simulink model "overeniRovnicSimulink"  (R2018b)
settings: Solver=ode4  StartTime=0.0  StopTime=5  FixedStep=1e-3  RelTol=1e-3
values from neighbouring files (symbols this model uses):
  b_0 = 0    [mainSkript_overeniRovnic.m]    (also in mainSkript_rovniceSystemu.m = (params.bp_0 + params.bn_0) / 2; mainSkript_simulaceLQG.m = (bn_0 + bp_0) / 2; mainSkript_LQGexperiment.m = (bn_0 + bp_0) / 2; mainSkript_LQGexperiment_integral.m = (bn_0 + bp_0) / 2)
  b_1 = params.b_1    [mainSkript_overeniRovnic.m]    (also in mainSkript_rovniceSystemu.m; mainSkript_kyvadlaNajednouOdhad.m; mainSkript_simulaceLQG.m; mainSkript_LQGexperiment.m)
  b_2 = params.b_2    [mainSkript_overeniRovnic.m]    (also in mainSkript_rovniceSystemu.m; mainSkript_kyvadlaNajednouOdhad.m; mainSkript_simulaceLQG.m; mainSkript_LQGexperiment.m)
  dtheta0_0 = 0    [mainSkript_overeniRovnic.m]
  dtheta0_1 = 0    [mainSkript_overeniRovnic.m]    (also in mainSkript_kyvadlaNajednouOdhad.m = filt * dth1(n_start-gl : n_start+gl))
  dtheta0_2 = 0    [mainSkript_overeniRovnic.m]    (also in mainSkript_kyvadlaNajednouOdhad.m = filt * dth2(n_start-gl : n_start+gl))
  g = 9.81    [mainSkript_overeniRovnic.m]    (also in mainSkript_rovniceSystemu.m; mainSkript_estimaceVozik.m; mainSkript_odhadKyvadlaZvlast.m; mainSkript_kyvadlaNajednouOdhad.m)
  I_1 = params.I_1    [mainSkript_overeniRovnic.m]    (also in mainSkript_rovniceSystemu.m; mainSkript_kyvadlaNajednouOdhad.m; mainSkript_simulaceLQG.m; mainSkript_LQGexperiment.m)
  I_2 = params.I_2    [mainSkript_overeniRovnic.m]    (also in mainSkript_rovniceSystemu.m; mainSkript_kyvadlaNajednouOdhad.m; mainSkript_simulaceLQG.m; mainSkript_LQGexperiment.m)
  L_1 = params.L_1    [mainSkript_overeniRovnic.m]    (also in mainSkript_rovniceSystemu.m; odhadovane_parametry.m = 0.228; mainSkript_kyvadlaNajednouOdhad.m; mainSkript_simulaceLQG.m)
  l_1 = params.l_1    [mainSkript_overeniRovnic.m]    (also in mainSkript_rovniceSystemu.m; odhadovane_parametry.m = 0.134; mainSkript_kyvadlaNajednouOdhad.m; mainSkript_simulaceLQG.m)
  l_2 = params.l_2    [mainSkript_overeniRovnic.m]    (also in mainSkript_rovniceSystemu.m; odhadovane_parametry.m = 0.112; mainSkript_kyvadlaNajednouOdhad.m; mainSkript_simulaceLQG.m)
  m = params.m_0    [mainSkript_estimaceVozik.m]    (also in mainSkript_odhadKyvadlaZvlast.m = params.m_2; mainSkript_modifikaceVozik.m = 1.437)
  m_0 = params.m_0    [mainSkript_overeniRovnic.m]    (also in mainSkript_rovniceSystemu.m; mainSkript_simulaceLQG.m; mainSkript_LQGexperiment.m; mainSkript_LQGexperiment_integral.m)
  m_1 = params.m_1    [mainSkript_overeniRovnic.m]    (also in mainSkript_rovniceSystemu.m; mainSkript_kyvadlaNajednouOdhad.m; mainSkript_simulaceLQG.m; mainSkript_LQGexperiment.m)
  m_2 = params.m_2    [mainSkript_overeniRovnic.m]    (also in mainSkript_rovniceSystemu.m; mainSkript_kyvadlaNajednouOdhad.m; mainSkript_simulaceLQG.m; mainSkript_LQGexperiment.m)
  N = N * Cref'    [mainSkript_simulaceLQG.m]    (also in mainSkript_tvorbaTrajektorii.m = 100; mainSkript_pocitaniTVLQR_simplified.m = floor( length(time) / krok ))
  theta0_0 = 0    [mainSkript_overeniRovnic.m]
  theta0_1 = 0.1    [mainSkript_overeniRovnic.m]
  theta0_2 = -0.6    [mainSkript_overeniRovnic.m]
undefined symbols (not defined in the file or in its folder): deg, DiscIntNeverNeededParam, kg, rad, s
libraries: mblibv1 x33, simulink x2
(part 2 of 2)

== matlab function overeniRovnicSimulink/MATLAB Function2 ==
function dx = PohybovaRceDIP_basic(y, u, g, m_0, m_1, m_2, I_1, I_2, l_1, l_2, L_1, b_0, b_1, b_2)
%PohybovaRceDIP_basic: Pohybova rovnice dvojiteho kyvadla

dx = zeros(6, 1); % definovani sloupcoveho vektoru derivaci stavu 

dx(1) = conj(y(4)); 
dx(2) = conj(y(5)); 
dx(3) = conj(y(6)); 
dx(4) = conj(y(6))*((b_2*(L_1^2*l_2*m_2^2*cos(y(3)) + I_1*l_2*m_2*cos(y(3)) - L_1^2*l_2*m_2^2*cos(y(2) - y(3))*cos(y(2)) + l_1^2*l_2*m_1*m_2*cos(y(3)) - L_1*l_1*l_2*m_1*m_2*cos(y(2) - y(3))*cos(y(2))))/(I_2*L_1^2*m_2^2 + I_2*l_1^2*m_1^2 + I_1*l_2^2*m_2^2 + I_1*I_2*m_0 + I_1*I_2*m_1 + I_1*I_2*m_2 + L_1^2*l_2^2*m_2^3 + L_1^2*l_2^2*m_0*m_2^2 + L_1^2*l_2^2*m_1*m_2^2 - L_1^2*l_2^2*m_2^3*cos(y(2) - y(3))^2 + I_2*L_1^2*m_0*m_2 + I_2*L_1^2*m_1*m_2 + l_1^2*l_2^2*m_1*m_2^2 + l_1^2*l_2^2*m_1^2*m_2 + I_2*l_1^2*m_0*m_1 + I_1*l_2^2*m_0*m_2 + I_1*l_2^2*m_1*m_2 + I_2*l_1^2*m_1*m_2 - I_2*L_1^2*m_2^2*cos(y(2))^2 - I_2*l_1^2*m_1^2*cos(y(2))^2 - I_1*l_2^2*m_2^2*cos(y(3))^2 - L_1^2*l_2^2*m_2^3*cos(y(2))^2 - L_1^2*l_2^2*m_2^3*cos(y(3))^2 + l_1^2*l_2^2*m_0*m_1*m_2 - l_1^2*l_2^2*m_1^2*m_2*cos(y(2))^2 - l_1^2*l_2^2*m_1*m_2^2*cos(y(3))^2 - L_1^2*l_2^2*m_0*m_2^2*cos(y(2) - y(3))^2 - L_1^2*l_2^2*m_1*m_2^2*cos(y(2) - y(3))^2 - 2*L_1*l_1*l_2^2*m_1*m_2^2*cos(y(2))^2 + 2*L_1^2*l_2^2*m_2^3*cos(y(2) - y(3))*cos(y(2))*cos(y(3)) - 2*I_2*L_1*l_1*m_1*m_2*cos(y(2))^2 + 2*L_1*l_1*l_2^2*m_1*m_2^2*cos(y(2) - y(3))*cos(y(2))*cos(y(3))) - ((b_2 - L_1*l_2*m_2*sin(y(2) - y(3))*y(6))*(L_1*l_2^2*m_2^2*cos(y(2)) + I_2*L_1*m_2*cos(y(2)) + I_2*l_1*m_1*cos(y(2)) - L_1*l_2^2*m_2^2*cos(y(2) - y(3))*cos(y(3)) + l_1*l_2^2*m_1*m_2*cos(y(2))))/(I_2*L_1^2*m_2^2 + I_2*l_1^2*m_1^2 + I_1*l_2^2*m_2^2 + I_1*I_2*m_0 + I_1*I_2*m_1 + I_1*I_2*m_2 + L_1^2*l_2^2*m_2^3 + L_1^2*l_2^2*m_0*m_2^2 + L_1^2*l_2^2*m_1*m_2^2 - L_1^2*l_2^2*m_2^3*cos(y(2) - y(3))^2 + I_2*L_1^2*m_0*m_2 + I_2*L_1^2*m_1*m_2 + l_1^2*l_2^2*m_1*m_2^2 + l_1^2*l_2^2*m_1^2*m_2 + I_2*l_1^2*m_0*m_1 + I_1*l_2^2*m_0*m_2 + I_1*l_2^2*m_1*m_2 + I_2*l_1^2*m_1*m_2 - I_2*L_1^2*m_2^2*cos(y(2))^2 - I_2*l_1^2*m_1^2*cos(y(2))^2 - I_1*l_2^2*m_2^2*cos(y(3))^2 - L_1^2*l_2^2*m_2^3*cos(y(2))^2 - L_1^2*l_2^2*m_2^3*cos(y(3))^2 + l_1^2*l_2^2*m_0*m_1*m_2 - l_1^2*l_2^2*m_1^2*m_2*cos(y(2))^2 - l_1^2*l_2^2*m_1*m_2^2*cos(y(3))^2 - L_1^2*l_2^2*m_0*m_2^2*cos(y(2) - y(3))^2 - L_1^2*l_2^2*m_1*m_2^2*cos(y(2) - y(3))^2 - 2*L_1*l_1*l_2^2*m_1*m_2^2*cos(y(2))^2 + 2*L_1^2*l_2^2*m_2^3*cos(y(2) - y(3))*cos(y(2))*cos(y(3)) - 2*I_2*L_1*l_1*m_1*m_2*cos(y(2))^2 + 2*L_1*l_1*l_2^2*m_1*m_2^2*cos(y(2) - y(3))*cos(y(2))*cos(y(3))) + (l_2*m_2*y(6)*sin(y(3))*(I_1*I_2 + L_1^2*l_2^2*m_2^2 + I_2*L_1^2*m_2 + I_2*l_1^2*m_1 + I_1*l_2^2*m_2 - L_1^2*l_2^2*m_2^2*cos(y(2) - y(3))^2 + l_1^2*l_2^2*m_1*m_2))/(I_2*L_1^2*m_2^2 + I_2*l_1^2*m_1^2 + I_1*l_2^2*m_2^2 + I_1*I_2*m_0 + I_1*I_2*m_1 + I_1*I_2*m_2 + L_1^2*l_2^2*m_2^3 + L_1^2*l_2^2*m_0*m_2^2 + L_1^2*l_2^2*m_1*m_2^2 - L_1^2*l_2^2*m_2^3*cos(y(2) - y(3))^2 + I_2*L_1^2*m_0*m_2 + I_2*L_1^2*m_1*m_2 + l_1^2*l_2^2*m_1*m_2^2 + l_1^2*l_2^2*m_1^2*m_2 + I_2*l_1^2*m_0*m_1 + I_1*l_2^2*m_0*m_2 + I_1*l_2^2*m_1*m_2 + I_2*l_1^2*m_1*m_2 - I_2*L_1^2*m_2^2*cos(y(2))^2 - I_2*l_1^2*m_1^2*cos(y(2))^2 - I_1*l_2^2*m_2^2*cos(y(3))^2 - L_1^2*l_2^2*m_2^3*cos(y(2))^2 - L_1^2*l_2^2*m_2^3*cos(y(3))^2 + l_1^2*l_2^2*m_0*m_1*m_2 - l_1^2*l_2^2*m_1^2*m_2*cos(y(2))^2 - l_1^2*l_2^2*m_1*m_2^2*cos(y(3))^2 - L_1^2*l_2^2*m_0*m_2^2*cos(y(2) - y(3))^2 - L_1^2*l_2^2*m_1*m_2^2*cos(y(2) - y(3))^2 - 2*L_1*l_1*l_2^2*m_1*m_2^2*cos(y(2))^2 + 2*L_1^2*l_2^2*m_2^3*cos(y(2) - y(3))*cos(y(2))*cos(y(3)) - 2*I_2*L_1*l_1*m_1*m_2*cos(y(2))^2 + 2*L_1*l_1*l_2^2*m_1*m_2^2*cos(y(2) - y(3))*cos(y(2))*cos(y(3)))) + conj(y(5))*(((b_1 + b_2)*(L_1*l_2^2*m_2^2*cos(y(2)) + I_2*L_1*m_2*cos(y(2)) + I_2*l_1*m_1*cos(y(2)) - L_1*l_2^2*m_2^2*cos(y(2) - y(3))*cos(y(3)) + l_1*l_2^2*m_1*m_2*cos(y(2))))/(I_2*L_1^2*m_2^2 + I_2*l_1^2*m_1^2 + I_1*l_2^2*m_2^2 + I_1*I_2*m_0 + I_1*I_2*m_1 + I_1*I_2*m_2 + L_1^2*l_2^2*m_2^3 + L_1^2*l_2^2*m_0*m_2^2 + L_1^2*l_2^2*m_1*m_2^2 - L_1^2*l_2^2*m_2^3*cos(y(2) - y(3))^2 + I_2*L_1^2*m_0*m_2 + I_2*L_1^2*m_1*m_2 + l_1^2*l_2^2*m_1*m_2^2 + l_1^2*l_2^2*m_1^2*m_2 + I_2*l_1^2*m_0*m_1 + I_1*l_2^2*m_0*m_2 + I_1*l_2^2*m_1*m_2 + I_2*l_1^2*m_1*m_2 - I_2*L_1^2*m_2^2*cos(y(2))^2 - I_2*l_1^2*m_1^2*cos(y(2))^2 - I_1*l_2^2*m_2^2*cos(y(3))^2 - L_1^2*l_2^2*m_2^3*cos(y(2))^2 - L_1^2*l_2^2*m_2^3*cos(y(3))^2 + l_1^2*l_2^2*m_0*m_1*m_2 - l_1^2*l_2^2*m_1^2*m_2*cos(y(2))^2 - l_1^2*l_2^2*m_1*m_2^2*cos(y(3))^2 - L_1^2*l_2^2*m_0*m_2^2*cos(y(2) - y(3))^2 - L_1^2*l_2^2*m_1*m_2^2*cos(y(2) - y(3))^2 - 2*L_1*l_1*l_2^2*m_1*m_2^2*cos(y(2))^2 + 2*L_1^2*l_2^2*m_2^3*cos(y(2) - y(3))*cos(y(2))*cos(y(3)) - 2*I_2*L_1*l_1*m_1*m_2*cos(y(2))^2 + 2*L_1*l_1*l_2^2*m_1*m_2^2*cos(y(2) - y(3))*cos(y(2))*cos(y(3))) - ((b_2 + L_1*l_2*m_2*sin(y(2) - y(3))*y(5))*(L_1^2*l_2*m_2^2*cos(y(3)) + I_1*l_2*m_2*cos(y(3)) - L_1^2*l_2*m_2^2*cos(y(2) - y(3))*cos(y(2)) + l_1^2*l_2*m_1*m_2*cos(y(3)) - L_1*l_1*l_2*m_1*m_2*cos(y(2) - y(3))*cos(y(2))))/(I_2*L_1^2*m_2^2 + I_2*l_1^2*m_1^2 + I_1*l_2^2*m_2^2 + I_1*I_2*m_0 + I_1*I_2*m_1 + I_1*I_2*m_2 + L_1^2*l_2^2*m_2^3 + L_1^2*l_2^2*m_0*m_2^2 + L_1^2*l_2^2*m_1*m_2^2 - L_1^2*l_2^2*m_2^3*cos(y(2) - y(3))^2 + I_2*L_1^2*m_0*m_2 + I_2*L_1^2*m_1*m_2 + l_1^2*l_2^2*m_1*m_2^2 + l_1^2*l_2^2*m_1^2*m_2 + I_2*l_1^2*m_0*m_1 + I_1*l_2^2*m_0*m_2 + I_1*l_2^2*m_1*m_2 + I_2*l_1^2*m_1*m_2 - I_2*L_1^2*m_2^2*cos(y(2))^2 - I_2*l_1^2*m_1^2*cos(y(2))^2 - I_1*l_2^2*m_2^2*cos(y(3))^2 - L_1^2*l_2^2*m_2^3*cos(y(2))^2 - L_1^2*l_2^2*m_2^3*cos(y(3))^2 + l_1^2*l_2^2*m_0*m_1*m_2 - l_1^2*l_2^2*m_1^2*m_2*cos(y(2))^2 - l_1^2*l_2^2*m_1*m_2^2*cos(y(3))^2 - L_1^2*l_2^2*m_0*m_2^2*cos(y(2) - y(3))^2 - L_1^2*l_2^2*m_1*m_2^2*cos(y(2) - y(3))^2 - 2*L_1*l_1*l_2^2*m_1*m_2^2*cos(y(2))^2 + 2*L_1^2*l_2^2*m_2^3*cos(y(2) - y(3))*cos(y(2))*cos(y(3)) - 2*I_2*L_1*l_1*m_1*m_2*cos(y(2))^2 + 2*L_1*l_1*l_2^2*m_1*m_2^2*cos(y(2) - y(3))*cos(y(2))*cos(y(3))) + (y(5)*sin(y(2))*(L_1*m_2 + l_1*m_1)*(I_1*I_2 + L_1^2*l_2^2*m_2^2 + I_2*L_1^2*m_2 + I_2*l_1^2*m_1 + I_1*l_2^2*m_2 - L_1^2*l_2^2*m_2^2*cos(y(2) - y(3))^2 + l_1^2*l_2^2*m_1*m_2))/(I_2*L_1^2*m_2^2 + I_2*l_1^2*m_1^2 + I_1*l_2^2*m_2^2 + I_1*I_2*m_0 + I_1*I_2*m_1 + I_1*I_2*m_2 + L_1^2*l_2^2*m_2^3 + L_1^2*l_2^2*m_0*m_2^2 + L_1^2*l_2^2*m_1*m_2^2 - L_1^2*l_2^2*m_2^3*cos(y(2) - y(3))^2 + I_2*L_1^2*m_0*m_2 + I_2*L_1^2*m_1*m_2 + l_1^2*l_2^2*m_1*m_2^2 + l_1^2*l_2^2*m_1^2*m_2 + I_2*l_1^2*m_0*m_1 + I_1*l_2^2*m_0*m_2 + I_1*l_2^2*m_1*m_2 + I_2*l_1^2*m_1*m_2 - I_2*L_1^2*m_2^2*cos(y(2))^2 - I_2*l_1^2*m_1^2*cos(y(2))^2 - I_1*l_2^2*m_2^2*cos(y(3))^2 - L_1^2*l_2^2*m_2^3*cos(y(2))^2 - L_1^2*l_2^2*m_2^3*cos(y(3))^2 + l_1^2*l_2^2*m_0*m_1*m_2 - l_1^2*l_2^2*m_1^2*m_2*cos(y(2))^2 - l_1^2*l_2^2*m_1*m_2^2*cos(y(3))^2 - L_1^2*l_2^2*m_0*m_2^2*cos(y(2) - y(3))^2 - L_1^2*l_2^2*m_1*m_2^2*cos(y(2) - y(3))^2 - 2*L_1*l_1*l_2^2*m_1*m_2^2*cos(y(2))^2 + 2*L_1^2*l_2^2*m_2^3*cos(y(2) - y(3))*cos(y(2))*cos(y(3)) - 2*I_2*L_1*l_1*m_1*m_2*cos(y(2))^2 + 2*L_1*l_1*l_2^2*m_1*m_2^2*cos(y(2) - y(3))*cos(y(2))*cos(y(3)))) + (u*(I_1*I_2 + L_1^2*l_2^2*m_2^2 + I_2*L_1^2*m_2 + I_2*l_1^2*m_1 + I_1*l_2^2*m_2 - L_1^2*l_2^2*m_2^2*cos(y(2) - y(3))^2 + l_1^2*l_2^2*m_1*m_2))/(I_2*L_1^2*m_2^2 + I_2*l_1^2*m_1^2 + I_1*l_2^2*m_2^2 + I_1*I_2*m_0 + I_1*I_2*m_1 + I_1*I_2*m_2 + L_1^2*l_2^2*m_2^3 + L_1^2*l_2^2*m_0*m_2^2 + L_1^2*l_2^2*m_1*m_2^2 - L_1^2*l_2^2*m_2^3*cos(y(2) - y(3))^2 + I_2*L_1^2*m_0*m_2 + I_2*L_1^2*m_1*m_2 + l_1^2*l_2^2*m_1*m_2^2 + l_1^2*l_2^2*m_1^2*m_2 + I_2*l_1^2*m_0*m_1 + I_1*l_2^2*m_0*m_2 + I_1*l_2^2*m_1*m_2 + I_2*l_1^2*m_1*m_2 - I_2*L_1^2*m_2^2*cos(y(2))^2 - I_2*l_1^2*m_1^2*cos(y(2))^2 - I_1*l_2^2*m_2^2*cos(y(3))^2 - L_1^2*l_2^2*m_2^3*cos(y(2))^2 - L_1^2*l_2^2*m_2^3*cos(y(3))^2 + l_1^2*l_2^2*m_0*m_1*m_2 - l_1^2*l_2^2*m_1^2*m_2*cos(y(2))^2 - l_1^2*l_2^2*m_1*m_2^2*cos(y(3))^2 - L_1^2*l_2^2*m_0*m_2^2*cos(y(2) - y(3))^2 - L_1^2*l_2^2*m_1*m_2^2*cos(y(2) - y(3))^2 - 2*L_1*l_1*l_2^2*m_1*m_2^2*cos(y(2))^2 + 2*L_1^2*l_2^2*m_2^3*cos(y(2) - y(3))*cos(y(2))*cos(y(3)) - 2*I_2*L_1*l_1*m_1*m_2*cos(y(2))^2 + 2*L_1*l_1*l_2^2*m_1*m_2^2*cos(y(2) - y(3))*cos(y(2))*cos(y(3))) - (b_0*conj(y(4))*(I_1*I_2 + L_1^2*l_2^2*m_2^2 + I_2*L_1^2*m_2 + I_2*l_1^2*m_1 + I_1*l_2^2*m_2 - L_1^2*l_2^2*m_2^2*cos(y(2) - y(3))^2 + l_1^2*l_2^2*m_1*m_2))/(I_2*L_1^2*m_2^2 + I_2*l_1^2*m_1^2 + I_1*l_2^2*m_2^2 + I_1*I_2*m_0 + I_1*I_2*m_1 + I_1*I_2*m_2 + L_1^2*l_2^2*m_2^3 + L_1^2*l_2^2*m_0*m_2^2 + L_1^2*l_2^2*m_1*m_2^2 - L_1^2*l_2^2*m_2^3*cos(y(2) - y(3))^2 + I_2*L_1^2*m_0*m_2 + I_2*L_1^2*m_1*m_2 + l_1^2*l_2^2*m_1*m_2^2 + l_1^2*l_2^2*m_1^2*m_2 + I_2*l_1^2*m_0*m_1 + I_1*l_2^2*m_0*m_2 + I_1*l_2^2*m_1*m_2 + I_2*l_1^2*m_1*m_2 - I_2*L_1^2*m_2^2*cos(y(2))^2 - I_2*l_1^2*m_1^2*cos(y(2))^2 - I_1*l_2^2*m_2^2*cos(y(3))^2 - L_1^2*l_2^2*m_2^3*cos(y(2))^2 - L_1^2*l_2^2*m_2^3*cos(y(3))^2 + l_1^2*l_2^2*m_0*m_1*m_2 - l_1^2*l_2^2*m_1^2*m_2*cos(y(2))^2 - l_1^2*l_2^2*m_1*m_2^2*cos(y(3))^2 - L_1^2*l_2^2*m_0*m_2^2*cos(y(2) - y(3))^2 - L_1^2*l_2^2*m_1*m_2^2*cos(y(2) - y(3))^2 - 2*L_1*l_1*l_2^2*m_1*m_2^2*cos(y(2))^2 + 2*L_1^2*l_2^2*m_2^3*cos(y(2) - y(3))*cos(y(2))*cos(y(3)) - 2*I_2*L_1*l_1*m_1*m_2*cos(y(2))^2 + 2*L_1*l_1*l_2^2*m_1*m_2^2*cos(y(2) - y(3))*cos(y(2))*cos(y(3))) - (g*sin(y(2))*(L_1*m_2 + l_1*m_1)*(L_1*l_2^2*m_2^2*cos(y(2)) + I_2*L_1*m_2*cos(y(2)) + I_2*l_1*m_1*cos(y(2)) - L_1*l_2^2*m_2^2*cos(y(2) - y(3))*cos(y(3)) + l_1*l_2^2*m_1*m_2*cos(y(2))))/(I_2*L_1^2*m_2^2 + I_2*l_1^2*m_1^2 + I_1*l_2^2*m_2^2 + I_1*I_2*m_0 + I_1*I_2*m_1 + I_1*I_2*m_2 + L_1^2*l_2^2*m_2^3 + L_1^2*l_2^2*m_0*m_2^2 + L_1^2*l_2^2*m_1*m_2^2 - L_1^2*l_2^2*m_2^3*cos(y(2) - y(3))^2 + I_2*L_1^2*m_0*m_2 + I_2*L_1^2*m_1*m_2 + l_1^2*l_2^2*m_1*m_2^2 + l_1^2*l_2^2*m_1^2*m_2 + I_2*l_1^2*m_0*m_1 + I_1*l_2^2*m_0*m_2 + I_1*l_2^2*m_1*m_2 + I_2*l_1^2*m_1*m_2 - I_2*L_1^2*m_2^2*cos(y(2))^2 - I_2*l_1^2*m_1^2*cos(y(2))^2 - I_1*l_2^2*m_2^2*cos(y(3))^2 - L_1^2*l_2^2*m_2^3*cos(y(2))^2 - L_1^2*l_2^2*m_2^3*cos(y(3))^2 + l_1^2*l_2^2*m_0*m_1*m_2 - l_1^2*l_2^2*m_1^2*m_2*cos(y(2))^2 - l_1^2*l_2^2*m_1*m_2^2*cos(y(3))^2 - L_1^2*l_2^2*m_0*m_2^2*cos(y(2) - y(3))^2 - L_1^2*l_2^2*m_1*m_2^2*cos(y(2) - y(3))^2 - 2*L_1*l_1*l_2^2*m_1*m_2^2*cos(y(2))^2 + 2*L_1^2*l_2^2*m_2^3*cos(y(2) - y(3))*cos(y(2))*cos(y(3)) - 2*I_2*L_1*l_1*m_1*m_2*cos(y(2))^2 + 2*L_1*l_1*l_2^2*m_1*m_2^2*cos(y(2) - y(3))*cos(y(2))*cos(y(3))) - (g*l_2*m_2*sin(y(3))*(L_1^2*l_2*m_2^2*cos(y(3)) + I_1*l_2*m_2*cos(y(3)) - L_1^2*l_2*m_2^2*cos(y(2) - y(3))*cos(y(2)) + l_1^2*l_2*m_1*m_2*cos(y(3)) - L_1*l_1*l_2*m_1*m_2*cos(y(2) - y(3))*cos(y(2))))/(I_2*L_1^2*m_2^2 + I_2*l_1^2*m_1^2 + I_1*l_2^2*m_2^2 + I_1*I_2*m_0 + I_1*I_2*m_1 + I_1*I_2*m_2 + L_1^2*l_2^2*m_2^3 + L_1^2*l_2^2*m_0*m_2^2 + L_1^2*l_2^2*m_1*m_2^2 - L_1^2*l_2^2*m_2^3*cos(y(2) - y(3))^2 + I_2*L_1^2*m_0*m_2 + I_2*L_1^2*m_1*m_2 + l_1^2*l_2^2*m_1*m_2^2 + l_1^2*l_2^2*m_1^2*m_2 + I_2*l_1^2*m_0*m_1 + I_1*l_2^2*m_0*m_2 + I_1*l_2^2*m_1*m_2 + I_2*l_1^2*m_1*m_2 - I_2*L_1^2*m_2^2*cos(y(2))^2 - I_2*l_1^2*m_1^2*cos(y(2))^2 - I_1*l_2^2*m_2^2*cos(y(3))^2 - L_1^2*l_2^2*m_2^3*cos(y(2))^2 - L_1^2*l_2^2*m_2^3*cos(y(3))^2 + l_1^2*l_2^2*m_0*m_1*m_2 - l_1^2*l_2^2*m_1^2*m_2*cos(y(2))^2 - l_1^2*l_2^2*m_1*m_2^2*cos(y(3))^2 - L_1^2*l_2^2*m_0*m_2^2*cos(y(2) - y(3))^2 - L_1^2*l_2^2*m_1*m_2^2*cos(y(2) - y(3))^2 - 2*L_1*l_1*l_2^2*m_1*m_2^2*cos(y(2))^2 + 2*L_1^2*l_2^2*m_2^3*cos(y(2) - y(3))*cos(y(2))*cos(y(3)) - 2*I_2*L_1*l_1*m_1*m_2*cos(y(2))^2 + 2*L_1*l_1*l_2^2*m_1*m_2^2*cos(y(2) - y(3))*cos(y(2))*cos(y(3))); 
dx(5) = conj(y(6))*((b_2*(L_1*l_2*m_2^2*cos(y(2) - y(3)) + L_1*l_2*m_0*m_2*cos(y(2) - y(3)) + L_1*l_2*m_1*m_2*cos(y(2) - y(3)) - L_1*l_2*m_2^2*cos(y(2))*cos(y(3)) - l_1*l_2*m_1*m_2*cos(y(2))*cos(y(3))))/(I_2*L_1^2*m_2^2 + I_2*l_1^2*m_1^2 + I_1*l_2^2*m_2^2 + I_1*I_2*m_0 + I_1*I_2*m_1 + I_1*I_2*m_2 + L_1^2*l_2^2*m_2^3 + L_1^2*l_2^2*m_0*m_2^2 + L_1^2*l_2^2*m_1*m_2^2 - L_1^2*l_2^2*m_2^3*cos(y(2) - y(3))^2 + I_2*L_1^2*m_0*m_2 + I_2*L_1^2*m_1*m_2 + l_1^2*l_2^2*m_1*m_2^2 + l_1^2*l_2^2*m_1^2*m_2 + I_2*l_1^2*m_0*m_1 + I_1*l_2^2*m_0*m_2 + I_1*l_2^2*m_1*m_2 + I_2*l_1^2*m_1*m_2 - I_2*L_1^2*m_2^2*cos(y(2))^2 - I_2*l_1^2*m_1^2*cos(y(2))^2 - I_1*l_2^2*m_2^2*cos(y(3))^2 - L_1^2*l_2^2*m_2^3*cos(y(2))^2 - L_1^2*l_2^2*m_2^3*cos(y(3))^2 + l_1^2*l_2^2*m_0*m_1*m_2 - l_1^2*l_2^2*m_1^2*m_2*cos(y(2))^2 - l_1^2*l_2^2*m_1*m_2^2*cos(y(3))^2 - L_1^2*l_2^2*m_0*m_2^2*cos(y(2) - y(3))^2 - L_1^2*l_2^2*m_1*m_2^2*cos(y(2) - y(3))^2 - 2*L_1*l_1*l_2^2*m_1*m_2^2*cos(y(2))^2 + 2*L_1^2*l_2^2*m_2^3*cos(y(2) - y(3))*cos(y(2))*cos(y(3)) - 2*I_2*L_1*l_1*m_1*m_2*cos(y(2))^2 + 2*L_1*l_1*l_2^2*m_1*m_2^2*cos(y(2) - y(3))*cos(y(2))*cos(y(3))) + ((b_2 - L_1*l_2*m_2*sin(y(2) - y(3))*y(6))*(I_2*m_0 + I_2*m_1 + I_2*m_2 + l_2^2*m_2^2 + l_2^2*m_0*m_2 + l_2^2*m_1*m_2 - l_2^2*m_2^2*cos(y(3))^2))/(I_2*L_1^2*m_2^2 + I_2*l_1^2*m_1^2 + I_1*l_2^2*m_2^2 + I_1*I_2*m_0 + I_1*I_2*m_1 + I_1*I_2*m_2 + L_1^2*l_2^2*m_2^3 + L_1^2*l_2^2*m_0*m_2^2 + L_1^2*l_2^2*m_1*m_2^2 - L_1^2*l_2^2*m_2^3*cos(y(2) - y(3))^2 + I_2*L_1^2*m_0*m_2 + I_2*L_1^2*m_1*m_2 + l_1^2*l_2^2*m_1*m_2^2 + l_1^2*l_2^2*m_1^2*m_2 + I_2*l_1^2*m_0*m_1 + I_1*l_2^2*m_0*m_2 + I_1*l_2^2*m_1*m_2 + I_2*l_1^2*m_1*m_2 - I_2*L_1^2*m_2^2*cos(y(2))^2 - I_2*l_1^2*m_1^2*cos(y(2))^2 - I_1*l_2^2*m_2^2*cos(y(3))^2 - L_1^2*l_2^2*m_2^3*cos(y(2))^2 - L_1^2*l_2^2*m_2^3*cos(y(3))^2 + l_1^2*l_2^2*m_0*m_1*m_2 - l_1^2*l_2^2*m_1^2*m_2*cos(y(2))^2 - l_1^2*l_2^2*m_1*m_2^2*cos(y(3))^2 - L_1^2*l_2^2*m_0*m_2^2*cos(y(2) - y(3))^2 - L_1^2*l_2^2*m_1*m_2^2*cos(y(2) - y(3))^2 - 2*L_1*l_1*l_2^2*m_1*m_2^2*cos(y(2))^2 + 2*L_1^2*l_2^2*m_2^3*cos(y(2) - y(3))*cos(y(2))*cos(y(3)) - 2*I_2*L_1*l_1*m_1*m_2*cos(y(2))^2 + 2*L_1*l_1*l_2^2*m_1*m_2^2*cos(y(2) - y(3))*cos(y(2))*cos(y(3))) - (l_2*m_2*y(6)*sin(y(3))*(L_1*l_2^2*m_2^2*cos(y(2)) + I_2*L_1*m_2*cos(y(2)) + I_2*l_1*m_1*cos(y(2)) - L_1*l_2^2*m_2^2*cos(y(2) - y(3))*cos(y(3)) + l_1*l_2^2*m_1*m_2*cos(y(2))))/(I_2*L_1^2*m_2^2 + I_2*l_1^2*m_1^2 + I_1*l_2^2*m_2^2 + I_1*I_2*m_0 + I_1*I_2*m_1 + I_1*I_2*m_2 + L_1^2*l_2^2*m_2^3 + L_1^2*l_2^2*m_0*m_2^2 + L_1^2*l_2^2*m_1*m_2^2 - L_1^2*l_2^2*m_2^3*cos(y(2) - y(3))^2 + I_2*L_1^2*m_0*m_2 + I_2*L_1^2*m_1*m_2 + l_1^2*l_2^2*m_1*m_2^2 + l_1^2*l_2^2*m_1^2*m_2 + I_2*l_1^2*m_0*m_1 + I_1*l_2^2*m_0*m_2 + I_1*l_2^2*m_1*m_2 + I_2*l_1^2*m_1*m_2 - I_2*L_1^2*m_2^2*cos(y(2))^2 - I_2*l_1^2*m_1^2*cos(y(2))^2 - I_1*l_2^2*m_2^2*cos(y(3))^2 - L_1^2*l_2^2*m_2^3*cos(y(2))^2 - L_1^2*l_2^2*m_2^3*cos(y(3))^2 + l_1^2*l_2^2*m_0*m_1*m_2 - l_1^2*l_2^2*m_1^2*m_2*cos(y(2))^2 - l_1^2*l_2^2*m_1*m_2^2*cos(y(3))^2 - L_1^2*l_2^2*m_0*m_2^2*cos(y(2) - y(3))^2 - L_1^2*l_2^2*m_1*m_2^2*cos(y(2) - y(3))^2 - 2*L_1*l_1*l_2^2*m_1*m_2^2*cos(y(2))^2 + 2*L_1^2*l_2^2*m_2^3*cos(y(2) - y(3))*cos(y(2))*cos(y(3)) - 2*I_2*L_1*l_1*m_1*m_2*cos(y(2))^2 + 2*L_1*l_1*l_2^2*m_1*m_2^2*cos(y(2) - y(3))*cos(y(2))*cos(y(3)))) - conj(y(5))*(((b_1 + b_2)*(I_2*m_0 + I_2*m_1 + I_2*m_2 + l_2^2*m_2^2 + l_2^2*m_0*m_2 + l_2^2*m_1*m_2 - l_2^2*m_2^2*cos(y(3))^2))/(I_2*L_1^2*m_2^2 + I_2*l_1^2*m_1^2 + I_1*l_2^2*m_2^2 + I_1*I_2*m_0 + I_1*I_2*m_1 + I_1*I_2*m_2 + L_1^2*l_2^2*m_2^3 + L_1^2*l_2^2*m_0*m_2^2 + L_1^2*l_2^2*m_1*m_2^2 - L_1^2*l_2^2*m_2^3*cos(y(2) - y(3))^2 + I_2*L_1^2*m_0*m_2 + I_2*L_1^2*m_1*m_2 + l_1^2*l_2^2*m_1*m_2^2 + l_1^2*l_2^2*m_1^2*m_2 + I_2*l_1^2*m_0*m_1 + I_1*l_2^2*m_0*m_2 + I_1*l_2^2*m_1*m_2 + I_2*l_1^2*m_1*m_2 - I_2*L_1^2*m_2^2*cos(y(2))^2 - I_2*l_1^2*m_1^2*cos(y(2))^2 - I_1*l_2^2*m_2^2*cos(y(3))^2 - L_1^2*l_2^2*m_2^3*cos(y(2))^2 - L_1^2*l_2^2*m_2^3*cos(y(3))^2 + l_1^2*l_2^2*m_0*m_1*m_2 - l_1^2*l_2^2*m_1^2*m_2*cos(y(2))^2 - l_1^2*l_2^2*m_1*m_2^2*cos(y(3))^2 - L_1^2*l_2^2*m_0*m_2^2*cos(y(2) - y(3))^2 - L_1^2*l_2^2*m_1*m_2^2*cos(y(2) - y(3))^2 - 2*L_1*l_1*l_2^2*m_1*m_2^2*cos(y(2))^2 + 2*L_1^2*l_2^2*m_2^3*cos(y(2) - y(3))*cos(y(2))*cos(y(3)) - 2*I_2*L_1*l_1*m_1*m_2*cos(y(2))^2 + 2*L_1*l_1*l_2^2*m_1*m_2^2*cos(y(2) - y(3))*cos(y(2))*cos(y(3))) + ((b_2 + L_1*l_2*m_2*sin(y(2) - y(3))*y(5))*(L_1*l_2*m_2^2*cos(y(2) - y(3)) + L_1*l_2*m_0*m_2*cos(y(2) - y(3)) + L_1*l_2*m_1*m_2*cos(y(2) - y(3)) - L_1*l_2*m_2^2*cos(y(2))*cos(y(3)) - l_1*l_2*m_1*m_2*cos(y(2))*cos(y(3))))/(I_2*L_1^2*m_2^2 + I_2*l_1^2*m_1^2 + I_1*l_2^2*m_2^2 + I_1*I_2*m_0 + I_1*I_2*m_1 + I_1*I_2*m_2 + L_1^2*l_2^2*m_2^3 + L_1^2*l_2^2*m_0*m_2^2 + L_1^2*l_2^2*m_1*m_2^2 - L_1^2*l_2^2*m_2^3*cos(y(2) - y(3))^2 + I_2*L_1^2*m_0*m_2 + I_2*L_1^2*m_1*m_2 + l_1^2*l_2^2*m_1*m_2^2 + l_1^2*l_2^2*m_1^2*m_2 + I_2*l_1^2*m_0*m_1 + I_1*l_2^2*m_0*m_2 + I_1*l_2^2*m_1*m_2 + I_2*l_1^2*m_1*m_2 - I_2*L_1^2*m_2^2*cos(y(2))^2 - I_2*l_1^2*m_1^2*cos(y(2))^2 - I_1*l_2^2*m_2^2*cos(y(3))^2 - L_1^2*l_2^2*m_2^3*cos(y(2))^2 - L_1^2*l_2^2*m_2^3*cos(y(3))^2 + l_1^2*l_2^2*m_0*m_1*m_2 - l_1^2*l_2^2*m_1^2*m_2*cos(y(2))^2 - l_1^2*l_2^2*m_1*m_2^2*cos(y(3))^2 - L_1^2*l_2^2*m_0*m_2^2*cos(y(2) - y(3))^2 - L_1^2*l_2^2*m_1*m_2^2*cos(y(2) - y(3))^2 - 2*L_1*l_1*l_2^2*m_1*m_2^2*cos(y(2))^2 + 2*L_1^2*l_2^2*m_2^3*cos(y(2) - y(3))*cos(y(2))*cos(y(3)) - 2*I_2*L_1*l_1*m_1*m_2*cos(y(2))^2 + 2*L_1*l_1*l_2^2*m_1*m_2^2*cos(y(2) - y(3))*cos(y(2))*cos(y(3))) + (y(5)*sin(y(2))*(L_1*m_2 + l_1*m_1)*(L_1*l_2^2*m_2^2*cos(y(2)) + I_2*L_1*m_2*cos(y(2)) + I_2*l_1*m_1*cos(y(2)) - L_1*l_2^2*m_2^2*cos(y(2) - y(3))*cos(y(3)) + l_1*l_2^2*m_1*m_2*cos(y(2))))/(I_2*L_1^2*m_2^2 + I_2*l_1^2*m_1^2 + I_1*l_2^2*m_2^2 + I_1*I_2*m_0 + I_1*I_2*m_1 + I_1*I_2*m_2 + L_1^2*l_2^2*m_2^3 + L_1^2*l_2^2*m_0*m_2^2 + L_1^2*l_2^2*m_1*m_2^2 - L_1^2*l_2^2*m_2^3*cos(y(2) - y(3))^2 + I_2*L_1^2*m_0*m_2 + I_2*L_1^2*m_1*m_2 + l_1^2*l_2^2*m_1*m_2^2 + l_1^2*l_2^2*m_1^2*m_2 + I_2*l_1^2*m_0*m_1 + I_1*l_2^2*m_0*m_2 + I_1*l_2^2*m_1*m_2 + I_2*l_1^2*m_1*m_2 - I_2*L_1^2*m_2^2*cos(y(2))^2 - I_2*l_1^2*m_1^2*cos(y(2))^2 - I_1*l_2^2*m_2^2*cos(y(3))^2 - L_1^2*l_2^2*m_2^3*cos(y(2))^2 - L_1^2*l_2^2*m_2^3*cos(y(3))^2 + l_1^2*l_2^2*m_0*m_1*m_2 - l_1^2*l_2^2*m_1^2*m_2*cos(y(2))^2 - l_1^2*l_2^2*m_1*m_2^2*cos(y(3))^2 - L_1^2*l_2^2*m_0*m_2^2*cos(y(2) - y(3))^2 - L_1^2*l_2^2*m_1*m_2^2*cos(y(2) - y(3))^2 - 2*L_1*l_1*l_2^2*m_1*m_2^2*cos(y(2))^2 + 2*L_1^2*l_2^2*m_2^3*cos(y(2) - y(3))*cos(y(2))*cos(y(3)) - 2*I_2*L_1*l_1*m_1*m_2*cos(y(2))^2 + 2*L_1*l_1*l_2^2*m_1*m_2^2*cos(y(2) - y(3))*cos(y(2))*cos(y(3)))) - (u*(L_1*l_2^2*m_2^2*cos(y(2)) + I_2*L_1*m_2*cos(y(2)) + I_2*l_1*m_1*cos(y(2)) - L_1*l_2^2*m_2^2*cos(y(2) - y(3))*cos(y(3)) + l_1*l_2^2*m_1*m_2*cos(y(2))))/(I_2*L_1^2*m_2^2 + I_2*l_1^2*m_1^2 + I_1*l_2^2*m_2^2 + I_1*I_2*m_0 + I_1*I_2*m_1 + I_1*I_2*m_2 + L_1^2*l_2^2*m_2^3 + L_1^2*l_2^2*m_0*m_2^2 + L_1^2*l_2^2*m_1*m_2^2 - L_1^2*l_2^2*m_2^3*cos(y(2) - y(3))^2 + I_2*L_1^2*m_0*m_2 + I_2*L_1^2*m_1*m_2 + l_1^2*l_2^2*m_1*m_2^2 + l_1^2*l_2^2*m_1^2*m_2 + I_2*l_1^2*m_0*m_1 + I_1*l_2^2*m_0*m_2 + I_1*l_2^2*m_1*m_2 + I_2*l_1^2*m_1*m_2 - I_2*L_1^2*m_2^2*cos(y(2))^2 - I_2*l_1^2*m_1^2*cos(y(2))^2 - I_1*l_2^2*m_2^2*cos(y(3))^2 - L_1^2*l_2^2*m_2^3*cos(y(2))^2 - L_1^2*l_2^2*m_2^3*cos(y(3))^2 + l_1^2*l_2^2*m_0*m_1*m_2 - l_1^2*l_2^2*m_1^2*m_2*cos(y(2))^2 - l_1^2*l_2^2*m_1*m_2^2*cos(y(3))^2 - L_1^2*l_2^2*m_0*m_2^2*cos(y(2) - y(3))^2 - L_1^2*l_2^2*m_1*m_2^2*cos(y(2) - y(3))^2 - 2*L_1*l_1*l_2^2*m_1*m_2^2*cos(y(2))^2 + 2*L_1^2*l_2^2*m_2^3*cos(y(2) - y(3))*cos(y(2))*cos(y(3)) - 2*I_2*L_1*l_1*m_1*m_2*cos(y(2))^2 + 2*L_1*l_1*l_2^2*m_1*m_2^2*cos(y(2) - y(3))*cos(y(2))*cos(y(3))) + (b_0*conj(y(4))*(L_1*l_2^2*m_2^2*cos(y(2)) + I_2*L_1*m_2*cos(y(2)) + I_2*l_1*m_1*cos(y(2)) - L_1*l_2^2*m_2^2*cos(y(2) - y(3))*cos(y(3)) + l_1*l_2^2*m_1*m_2*cos(y(2))))/(I_2*L_1^2*m_2^2 + I_2*l_1^2*m_1^2 + I_1*l_2^2*m_2^2 + I_1*I_2*m_0 + I_1*I_2*m_1 + I_1*I_2*m_2 + L_1^2*l_2^2*m_2^3 + L_1^2*l_2^2*m_0*m_2^2 + L_1^2*l_2^2*m_1*m_2^2 - L_1^2*l_2^2*m_2^3*cos(y(2) - y(3))^2 + I_2*L_1^2*m_0*m_2 + I_2*L_1^2*m_1*m_2 + l_1^2*l_2^2*m_1*m_2^2 + l_1^2*l_2^2*m_1^2*m_2 + I_2*l_1^2*m_0*m_1 + I_1*l_2^2*m_0*m_2 + I_1*l_2^2*m_1*m_2 + I_2*l_1^2*m_1*m_2 - I_2*L_1^2*m_2^2*cos(y(2))^2 - I_2*l_1^2*m_1^2*cos(y(2))^2 - I_1*l_2^2*m_2^2*cos(y(3))^2 - L_1^2*l_2^2*m_2^3*cos(y(2))^2 - L_1^2*l_2^2*m_2^3*cos(y(3))^2 + l_1^2*l_2^2*m_0*m_1*m_2 - l_1^2*l_2^2*m_1^2*m_2*cos(y(2))^2 - l_1^2*l_2^2*m_1*m_2^2*cos(y(3))^2 - L_1^2*l_2^2*m_0*m_2^2*cos(y(2) - y(3))^2 - L_1^2*l_2^2*m_1*m_2^2*cos(y(2) - y(3))^2 - 2*L_1*l_1*l_2^2*m_1*m_2^2*cos(y(2))^2 + 2*L_1^2*l_2^2*m_2^3*cos(y(2) - y(3))*cos(y(2))*cos(y(3)) - 2*I_2*L_1*l_1*m_1*m_2*cos(y(2))^2 + 2*L_1*l_1*l_2^2*m_1*m_2^2*cos(y(2) - y(3))*cos(y(2))*cos(y(3))) + (g*sin(y(2))*(L_1*m_2 + l_1*m_1)*(I_2*m_0 + I_2*m_1 + I_2*m_2 + l_2^2*m_2^2 + l_2^2*m_0*m_2 + l_2^2*m_1*m_2 - l_2^2*m_2^2*cos(y(3))^2))/(I_2*L_1^2*m_2^2 + I_2*l_1^2*m_1^2 + I_1*l_2^2*m_2^2 + I_1*I_2*m_0 + I_1*I_2*m_1 + I_1*I_2*m_2 + L_1^2*l_2^2*m_2^3 + L_1^2*l_2^2*m_0*m_2^2 + L_1^2*l_2^2*m_1*m_2^2 - L_1^2*l_2^2*m_2^3*cos(y(2) - y(3))^2 + I_2*L_1^2*m_0*m_2 + I_2*L_1^2*m_1*m_2 + l_1^2*l_2^2*m_1*m_2^2 + l_1^2*l_2^2*m_1^2*m_2 + I_2*l_1^2*m_0*m_1 + I_1*l_2^2*m_0*m_2 + I_1*l_2^2*m_1*m_2 + I_2*l_1^2*m_1*m_2 - I_2*L_1^2*m_2^2*cos(y(2))^2 - I_2*l_1^2*m_1^2*cos(y(2))^2 - I_1*l_2^2*m_2^2*cos(y(3))^2 - L_1^2*l_2^2*m_2^3*cos(y(2))^2 - L_1^2*l_2^2*m_2^3*cos(y(3))^2 + l_1^2*l_2^2*m_0*m_1*m_2 - l_1^2*l_2^2*m_1^2*m_2*cos(y(2))^2 - l_1^2*l_2^2*m_1*m_2^2*cos(y(3))^2 - L_1^2*l_2^2*m_0*m_2^2*cos(y(2) - y(3))^2 - L_1^2*l_2^2*m_1*m_2^2*cos(y(2) - y(3))^2 - 2*L_1*l_1*l_2^2*m_1*m_2^2*cos(y(2))^2 + 2*L_1^2*l_2^2*m_2^3*cos(y(2) - y(3))*cos(y(2))*cos(y(3)) - 2*I_2*L_1*l_1*m_1*m_2*cos(y(2))^2 + 2*L_1*l_1*l_2^2*m_1*m_2^2*cos(y(2) - y(3))*cos(y(2))*cos(y(3))) - (g*l_2*m_2*sin(y(3))*(L_1*l_2*m_2^2*cos(y(2) - y(3)) + L_1*l_2*m_0*m_2*cos(y(2) - y(3)) + L_1*l_2*m_1*m_2*cos(y(2) - y(3)) - L_1*l_2*m_2^2*cos(y(2))*cos(y(3)) - l_1*l_2*m_1*m_2*cos(y(2))*cos(y(3))))/(I_2*L_1^2*m_2^2 + I_2*l_1^2*m_1^2 + I_1*l_2^2*m_2^2 + I_1*I_2*m_0 + I_1*I_2*m_1 + I_1*I_2*m_2 + L_1^2*l_2^2*m_2^3 + L_1^2*l_2^2*m_0*m_2^2 + L_1^2*l_2^2*m_1*m_2^2 - L_1^2*l_2^2*m_2^3*cos(y(2) - y(3))^2 + I_2*L_1^2*m_0*m_2 + I_2*L_1^2*m_1*m_2 + l_1^2*l_2^2*m_1*m_2^2 + l_1^2*l_2^2*m_1^2*m_2 + I_2*l_1^2*m_0*m_1 + I_1*l_2^2*m_0*m_2 + I_1*l_2^2*m_1*m_2 + I_2*l_1^2*m_1*m_2 - I_2*L_1^2*m_2^2*cos(y(2))^2 - I_2*l_1^2*m_1^2*cos(y(2))^2 - I_1*l_2^2*m_2^2*cos(y(3))^2 - L_1^2*l_2^2*m_2^3*cos(y(2))^2 - L_1^2*l_2^2*m_2^3*cos(y(3))^2 + l_1^2*l_2^2*m_0*m_1*m_2 - l_1^2*l_2^2*m_1^2*m_2*cos(y(2))^2 - l_1^2*l_2^2*m_1*m_2^2*cos(y(3))^2 - L_1^2*l_2^2*m_0*m_2^2*cos(y(2) - y(3))^2 - L_1^2*l_2^2*m_1*m_2^2*cos(y(2) - y(3))^2 - 2*L_1*l_1*l_2^2*m_1*m_2^2*cos(y(2))^2 + 2*L_1^2*l_2^2*m_2^3*cos(y(2) - y(3))*cos(y(2))*cos(y(3)) - 2*I_2*L_1*l_1*m_1*m_2*cos(y(2))^2 + 2*L_1*l_1*l_2^2*m_1*m_2^2*cos(y(2) - y(3))*cos(y(2))*cos(y(3))); 
dx(6) = conj(y(5))*(((b_1 + b_2)*(L_1*l_2*m_2^2*cos(y(2) - y(3)) + L_1*l_2*m_0*m_2*cos(y(2) - y(3)) + L_1*l_2*m_1*m_2*cos(y(2) - y(3)) - L_1*l_2*m_2^2*cos(y(2))*cos(y(3)) - l_1*l_2*m_1*m_2*cos(y(2))*cos(y(3))))/(I_2*L_1^2*m_2^2 + I_2*l_1^2*m_1^2 + I_1*l_2^2*m_2^2 + I_1*I_2*m_0 + I_1*I_2*m_1 + I_1*I_2*m_2 + L_1^2*l_2^2*m_2^3 + L_1^2*l_2^2*m_0*m_2^2 + L_1^2*l_2^2*m_1*m_2^2 - L_1^2*l_2^2*m_2^3*cos(y(2) - y(3))^2 + I_2*L_1^2*m_0*m_2 + I_2*L_1^2*m_1*m_2 + l_1^2*l_2^2*m_1*m_2^2 + l_1^2*l_2^2*m_1^2*m_2 + I_2*l_1^2*m_0*m_1 + I_1*l_2^2*m_0*m_2 + I_1*l_2^2*m_1*m_2 + I_2*l_1^2*m_1*m_2 - I_2*L_1^2*m_2^2*cos(y(2))^2 - I_2*l_1^2*m_1^2*cos(y(2))^2 - I_1*l_2^2*m_2^2*cos(y(3))^2 - L_1^2*l_2^2*m_2^3*cos(y(2))^2 - L_1^2*l_2^2*m_2^3*cos(y(3))^2 + l_1^2*l_2^2*m_0*m_1*m_2 - l_1^2*l_2^2*m_1^2*m_2*cos(y(2))^2 - l_1^2*l_2^2*m_1*m_2^2*cos(y(3))^2 - L_1^2*l_2^2*m_0*m_2^2*cos(y(2) - y(3))^2 - L_1^2*l_2^2*m_1*m_2^2*cos(y(2) - y(3))^2 - 2*L_1*l_1*l_2^2*m_1*m_2^2*cos(y(2))^2 + 2*L_1^2*l_2^2*m_2^3*cos(y(2) - y(3))*cos(y(2))*cos(y(3)) - 2*I_2*L_1*l_1*m_1*m_2*cos(y(2))^2 + 2*L_1*l_1*l_2^2*m_1*m_2^2*cos(y(2) - y(3))*cos(y(2))*cos(y(3))) + ((b_2 + L_1*l_2*m_2*sin(y(2) - y(3))*y(5))*(I_1*m_0 + I_1*m_1 + I_1*m_2 + L_1^2*m_2^2 + l_1^2*m_1^2 + l_1^2*m_0*m_1 + l_1^2*m_1*m_2 - L_1^2*m_2^2*cos(y(2))^2 - l_1^2*m_1^2*cos(y(2))^2 + L_1^2*m_0*m_2 + L_1^2*m_1*m_2 - 2*L_1*l_1*m_1*m_2*cos(y(2))^2))/(I_2*L_1^2*m_2^2 + I_2*l_1^2*m_1^2 + I_1*l_2^2*m_2^2 + I_1*I_2*m_0 + I_1*I_2*m_1 + I_1*I_2*m_2 + L_1^2*l_2^2*m_2^3 + L_1^2*l_2^2*m_0*m_2^2 + L_1^2*l_2^2*m_1*m_2^2 - L_1^2*l_2^2*m_2^3*cos(y(2) - y(3))^2 + I_2*L_1^2*m_0*m_2 + I_2*L_1^2*m_1*m_2 + l_1^2*l_2^2*m_1*m_2^2 + l_1^2*l_2^2*m_1^2*m_2 + I_2*l_1^2*m_0*m_1 + I_1*l_2^2*m_0*m_2 + I_1*l_2^2*m_1*m_2 + I_2*l_1^2*m_1*m_2 - I_2*L_1^2*m_2^2*cos(y(2))^2 - I_2*l_1^2*m_1^2*cos(y(2))^2 - I_1*l_2^2*m_2^2*cos(y(3))^2 - L_1^2*l_2^2*m_2^3*cos(y(2))^2 - L_1^2*l_2^2*m_2^3*cos(y(3))^2 + l_1^2*l_2^2*m_0*m_1*m_2 - l_1^2*l_2^2*m_1^2*m_2*cos(y(2))^2 - l_1^2*l_2^2*m_1*m_2^2*cos(y(3))^2 - L_1^2*l_2^2*m_0*m_2^2*cos(y(2) - y(3))^2 - L_1^2*l_2^2*m_1*m_2^2*cos(y(2) - y(3))^2 - 2*L_1*l_1*l_2^2*m_1*m_2^2*cos(y(2))^2 + 2*L_1^2*l_2^2*m_2^3*cos(y(2) - y(3))*cos(y(2))*cos(y(3)) - 2*I_2*L_1*l_1*m_1*m_2*cos(y(2))^2 + 2*L_1*l_1*l_2^2*m_1*m_2^2*cos(y(2) - y(3))*cos(y(2))*cos(y(3))) - (y(5)*sin(y(2))*(L_1*m_2 + l_1*m_1)*(L_1^2*l_2*m_2^2*cos(y(3)) + I_1*l_2*m_2*cos(y(3)) - L_1^2*l_2*m_2^2*cos(y(2) - y(3))*cos(y(2)) + l_1^2*l_2*m_1*m_2*cos(y(3)) - L_1*l_1*l_2*m_1*m_2*cos(y(2) - y(3))*cos(y(2))))/(I_2*L_1^2*m_2^2 + I_2*l_1^2*m_1^2 + I_1*l_2^2*m_2^2 + I_1*I_2*m_0 + I_1*I_2*m_1 + I_1*I_2*m_2 + L_1^2*l_2^2*m_2^3 + L_1^2*l_2^2*m_0*m_2^2 + L_1^2*l_2^2*m_1*m_2^2 - L_1^2*l_2^2*m_2^3*cos(y(2) - y(3))^2 + I_2*L_1^2*m_0*m_2 + I_2*L_1^2*m_1*m_2 + l_1^2*l_2^2*m_1*m_2^2 + l_1^2*l_2^2*m_1^2*m_2 + I_2*l_1^2*m_0*m_1 + I_1*l_2^2*m_0*m_2 + I_1*l_2^2*m_1*m_2 + I_2*l_1^2*m_1*m_2 - I_2*L_1^2*m_2^2*cos(y(2))^2 - I_2*l_1^2*m_1^2*cos(y(2))^2 - I_1*l_2^2*m_2^2*cos(y(3))^2 - L_1^2*l_2^2*m_2^3*cos(y(2))^2 - L_1^2*l_2^2*m_2^3*cos(y(3))^2 + l_1^2*l_2^2*m_0*m_1*m_2 - l_1^2*l_2^2*m_1^2*m_2*cos(y(2))^2 - l_1^2*l_2^2*m_1*m_2^2*cos(y(3))^2 - L_1^2*l_2^2*m_0*m_2^2*cos(y(2) - y(3))^2 - L_1^2*l_2^2*m_1*m_2^2*cos(y(2) - y(3))^2 - 2*L_1*l_1*l_2^2*m_1*m_2^2*cos(y(2))^2 + 2*L_1^2*l_2^2*m_2^3*cos(y(2) - y(3))*cos(y(2))*cos(y(3)) - 2*I_2*L_1*l_1*m_1*m_2*cos(y(2))^2 + 2*L_1*l_1*l_2^2*m_1*m_2^2*cos(y(2) - y(3))*cos(y(2))*cos(y(3)))) - conj(y(6))*((b_2*(I_1*m_0 + I_1*m_1 + I_1*m_2 + L_1^2*m_2^2 + l_1^2*m_1^2 + l_1^2*m_0*m_1 + l_1^2*m_1*m_2 - L_1^2*m_2^2*cos(y(2))^2 - l_1^2*m_1^2*cos(y(2))^2 + L_1^2*m_0*m_2 + L_1^2*m_1*m_2 - 2*L_1*l_1*m_1*m_2*cos(y(2))^2))/(I_2*L_1^2*m_2^2 + I_2*l_1^2*m_1^2 + I_1*l_2^2*m_2^2 + I_1*I_2*m_0 + I_1*I_2*m_1 + I_1*I_2*m_2 + L_1^2*l_2^2*m_2^3 + L_1^2*l_2^2*m_0*m_2^2 + L_1^2*l_2^2*m_1*m_2^2 - L_1^2*l_2^2*m_2^3*cos(y(2) - y(3))^2 + I_2*L_1^2*m_0*m_2 + I_2*L_1^2*m_1*m_2 + l_1^2*l_2^2*m_1*m_2^2 + l_1^2*l_2^2*m_1^2*m_2 + I_2*l_1^2*m_0*m_1 + I_1*l_2^2*m_0*m_2 + I_1*l_2^2*m_1*m_2 + I_2*l_1^2*m_1*m_2 - I_2*L_1^2*m_2^2*cos(y(2))^2 - I_2*l_1^2*m_1^2*cos(y(2))^2 - I_1*l_2^2*m_2^2*cos(y(3))^2 - L_1^2*l_2^2*m_2^3*cos(y(2))^2 - L_1^2*l_2^2*m_2^3*cos(y(3))^2 + l_1^2*l_2^2*m_0*m_1*m_2 - l_1^2*l_2^2*m_1^2*m_2*cos(y(2))^2 - l_1^2*l_2^2*m_1*m_2^2*cos(y(3))^2 - L_1^2*l_2^2*m_0*m_2^2*cos(y(2) - y(3))^2 - L_1^2*l_2^2*m_1*m_2^2*cos(y(2) - y(3))^2 - 2*L_1*l_1*l_2^2*m_1*m_2^2*cos(y(2))^2 + 2*L_1^2*l_2^2*m_2^3*cos(y(2) - y(3))*cos(y(2))*cos(y(3)) - 2*I_2*L_1*l_1*m_1*m_2*cos(y(2))^2 + 2*L_1*l_1*l_2^2*m_1*m_2^2*cos(y(2) - y(3))*cos(y(2))*cos(y(3))) + ((b_2 - L_1*l_2*m_2*sin(y(2) - y(3))*y(6))*(L_1*l_2*m_2^2*cos(y(2) - y(3)) + L_1*l_2*m_0*m_2*cos(y(2) - y(3)) + L_1*l_2*m_1*m_2*cos(y(2) - y(3)) - L_1*l_2*m_2^2*cos(y(2))*cos(y(3)) - l_1*l_2*m_1*m_2*cos(y(2))*cos(y(3))))/(I_2*L_1^2*m_2^2 + I_2*l_1^2*m_1^2 + I_1*l_2^2*m_2^2 + I_1*I_2*m_0 + I_1*I_2*m_1 + I_1*I_2*m_2 + L_1^2*l_2^2*m_2^3 + L_1^2*l_2^2*m_0*m_2^2 + L_1^2*l_2^2*m_1*m_2^2 - L_1^2*l_2^2*m_2^3*cos(y(2) - y(3))^2 + I_2*L_1^2*m_0*m_2 + I_2*L_1^2*m_1*m_2 + l_1^2*l_2^2*m_1*m_2^2 + l_1^2*l_2^2*m_1^2*m_2 + I_2*l_1^2*m_0*m_1 + I_1*l_2^2*m_0*m_2 + I_1*l_2^2*m_1*m_2 + I_2*l_1^2*m_1*m_2 - I_2*L_1^2*m_2^2*cos(y(2))^2 - I_2*l_1^2*m_1^2*cos(y(2))^2 - I_1*l_2^2*m_2^2*cos(y(3))^2 - L_1^2*l_2^2*m_2^3*cos(y(2))^2 - L_1^2*l_2^2*m_2^3*cos(y(3))^2 + l_1^2*l_2^2*m_0*m_1*m_2 - l_1^2*l_2^2*m_1^2*m_2*cos(y(2))^2 - l_1^2*l_2^2*m_1*m_2^2*cos(y(3))^2 - L_1^2*l_2^2*m_0*m_2^2*cos(y(2) - y(3))^2 - L_1^2*l_2^2*m_1*m_2^2*cos(y(2) - y(3))^2 - 2*L_1*l_1*l_2^2*m_1*m_2^2*cos(y(2))^2 + 2*L_1^2*l_2^2*m_2^3*cos(y(2) - y(3))*cos(y(2))*cos(y(3)) - 2*I_2*L_1*l_1*m_1*m_2*cos(y(2))^2 + 2*L_1*l_1*l_2^2*m_1*m_2^2*cos(y(2) - y(3))*cos(y(2))*cos(y(3))) + (l_2*m_2*y(6)*sin(y(3))*(L_1^2*l_2*m_2^2*cos(y(3)) + I_1*l_2*m_2*cos(y(3)) - L_1^2*l_2*m_2^2*cos(y(2) - y(3))*cos(y(2)) + l_1^2*l_2*m_1*m_2*cos(y(3)) - L_1*l_1*l_2*m_1*m_2*cos(y(2) - y(3))*cos(y(2))))/(I_2*L_1^2*m_2^2 + I_2*l_1^2*m_1^2 + I_1*l_2^2*m_2^2 + I_1*I_2*m_0 + I_1*I_2*m_1 + I_1*I_2*m_2 + L_1^2*l_2^2*m_2^3 + L_1^2*l_2^2*m_0*m_2^2 + L_1^2*l_2^2*m_1*m_2^2 - L_1^2*l_2^2*m_2^3*cos(y(2) - y(3))^2 + I_2*L_1^2*m_0*m_2 + I_2*L_1^2*m_1*m_2 + l_1^2*l_2^2*m_1*m_2^2 + l_1^2*l_2^2*m_1^2*m_2 + I_2*l_1^2*m_0*m_1 + I_1*l_2^2*m_0*m_2 + I_1*l_2^2*m_1*m_2 + I_2*l_1^2*m_1*m_2 - I_2*L_1^2*m_2^2*cos(y(2))^2 - I_2*l_1^2*m_1^2*cos(y(2))^2 - I_1*l_2^2*m_2^2*cos(y(3))^2 - L_1^2*l_2^2*m_2^3*cos(y(2))^2 - L_1^2*l_2^2*m_2^3*cos(y(3))^2 + l_1^2*l_2^2*m_0*m_1*m_2 - l_1^2*l_2^2*m_1^2*m_2*cos(y(2))^2 - l_1^2*l_2^2*m_1*m_2^2*cos(y(3))^2 - L_1^2*l_2^2*m_0*m_2^2*cos(y(2) - y(3))^2 - L_1^2*l_2^2*m_1*m_2^2*cos(y(2) - y(3))^2 - 2*L_1*l_1*l_2^2*m_1*m_2^2*cos(y(2))^2 + 2*L_1^2*l_2^2*m_2^3*cos(y(2) - y(3))*cos(y(2))*cos(y(3)) - 2*I_2*L_1*l_1*m_1*m_2*cos(y(2))^2 + 2*L_1*l_1*l_2^2*m_1*m_2^2*cos(y(2) - y(3))*cos(y(2))*cos(y(3)))) - (u*(L_1^2*l_2*m_2^2*cos(y(3)) + I_1*l_2*m_2*cos(y(3)) - L_1^2*l_2*m_2^2*cos(y(2) - y(3))*cos(y(2)) + l_1^2*l_2*m_1*m_2*cos(y(3)) - L_1*l_1*l_2*m_1*m_2*cos(y(2) - y(3))*cos(y(2))))/(I_2*L_1^2*m_2^2 + I_2*l_1^2*m_1^2 + I_1*l_2^2*m_2^2 + I_1*I_2*m_0 + I_1*I_2*m_1 + I_1*I_2*m_2 + L_1^2*l_2^2*m_2^3 + L_1^2*l_2^2*m_0*m_2^2 + L_1^2*l_2^2*m_1*m_2^2 - L_1^2*l_2^2*m_2^3*cos(y(2) - y(3))^2 + I_2*L_1^2*m_0*m_2 + I_2*L_1^2*m_1*m_2 + l_1^2*l_2^2*m_1*m_2^2 + l_1^2*l_2^2*m_1^2*m_2 + I_2*l_1^2*m_0*m_1 + I_1*l_2^2*m_0*m_2 + I_1*l_2^2*m_1*m_2 + I_2*l_1^2*m_1*m_2 - I_2*L_1^2*m_2^2*cos(y(2))^2 - I_2*l_1^2*m_1^2*cos(y(2))^2 - I_1*l_2^2*m_2^2*cos(y(3))^2 - L_1^2*l_2^2*m_2^3*cos(y(2))^2 - L_1^2*l_2^2*m_2^3*cos(y(3))^2 + l_1^2*l_2^2*m_0*m_1*m_2 - l_1^2*l_2^2*m_1^2*m_2*cos(y(2))^2 - l_1^2*l_2^2*m_1*m_2^2*cos(y(3))^2 - L_1^2*l_2^2*m_0*m_2^2*cos(y(2) - y(3))^2 - L_1^2*l_2^2*m_1*m_2^2*cos(y(2) - y(3))^2 - 2*L_1*l_1*l_2^2*m_1*m_2^2*cos(y(2))^2 + 2*L_1^2*l_2^2*m_2^3*cos(y(2) - y(3))*cos(y(2))*cos(y(3)) - 2*I_2*L_1*l_1*m_1*m_2*cos(y(2))^2 + 2*L_1*l_1*l_2^2*m_1*m_2^2*cos(y(2) - y(3))*cos(y(2))*cos(y(3))) + (b_0*conj(y(4))*(L_1^2*l_2*m_2^2*cos(y(3)) + I_1*l_2*m_2*cos(y(3)) - L_1^2*l_2*m_2^2*cos(y(2) - y(3))*cos(y(2)) + l_1^2*l_2*m_1*m_2*cos(y(3)) - L_1*l_1*l_2*m_1*m_2*cos(y(2) - y(3))*cos(y(2))))/(I_2*L_1^2*m_2^2 + I_2*l_1^2*m_1^2 + I_1*l_2^2*m_2^2 + I_1*I_2*m_0 + I_1*I_2*m_1 + I_1*I_2*m_2 + L_1^2*l_2^2*m_2^3 + L_1^2*l_2^2*m_0*m_2^2 + L_1^2*l_2^2*m_1*m_2^2 - L_1^2*l_2^2*m_2^3*cos(y(2) - y(3))^2 + I_2*L_1^2*m_0*m_2 + I_2*L_1^2*m_1*m_2 + l_1^2*l_2^2*m_1*m_2^2 + l_1^2*l_2^2*m_1^2*m_2 + I_2*l_1^2*m_0*m_1 + I_1*l_2^2*m_0*m_2 + I_1*l_2^2*m_1*m_2 + I_2*l_1^2*m_1*m_2 - I_2*L_1^2*m_2^2*cos(y(2))^2 - I_2*l_1^2*m_1^2*cos(y(2))^2 - I_1*l_2^2*m_2^2*cos(y(3))^2 - L_1^2*l_2^2*m_2^3*cos(y(2))^2 - L_1^2*l_2^2*m_2^3*cos(y(3))^2 + l_1^2*l_2^2*m_0*m_1*m_2 - l_1^2*l_2^2*m_1^2*m_2*cos(y(2))^2 - l_1^2*l_2^2*m_1*m_2^2*cos(y(3))^2 - L_1^2*l_2^2*m_0*m_2^2*cos(y(2) - y(3))^2 - L_1^2*l_2^2*m_1*m_2^2*cos(y(2) - y(3))^2 - 2*L_1*l_1*l_2^2*m_1*m_2^2*cos(y(2))^2 + 2*L_1^2*l_2^2*m_2^3*cos(y(2) - y(3))*cos(y(2))*cos(y(3)) - 2*I_2*L_1*l_1*m_1*m_2*cos(y(2))^2 + 2*L_1*l_1*l_2^2*m_1*m_2^2*cos(y(2) - y(3))*cos(y(2))*cos(y(3))) - (g*sin(y(2))*(L_1*m_2 + l_1*m_1)*(L_1*l_2*m_2^2*cos(y(2) - y(3)) + L_1*l_2*m_0*m_2*cos(y(2) - y(3)) + L_1*l_2*m_1*m_2*cos(y(2) - y(3)) - L_1*l_2*m_2^2*cos(y(2))*cos(y(3)) - l_1*l_2*m_1*m_2*cos(y(2))*cos(y(3))))/(I_2*L_1^2*m_2^2 + I_2*l_1^2*m_1^2 + I_1*l_2^2*m_2^2 + I_1*I_2*m_0 + I_1*I_2*m_1 + I_1*I_2*m_2 + L_1^2*l_2^2*m_2^3 + L_1^2*l_2^2*m_0*m_2^2 + L_1^2*l_2^2*m_1*m_2^2 - L_1^2*l_2^2*m_2^3*cos(y(2) - y(3))^2 + I_2*L_1^2*m_0*m_2 + I_2*L_1^2*m_1*m_2 + l_1^2*l_2^2*m_1*m_2^2 + l_1^2*l_2^2*m_1^2*m_2 + I_2*l_1^2*m_0*m_1 + I_1*l_2^2*m_0*m_2 + I_1*l_2^2*m_1*m_2 + I_2*l_1^2*m_1*m_2 - I_2*L_1^2*m_2^2*cos(y(2))^2 - I_2*l_1^2*m_1^2*cos(y(2))^2 - I_1*l_2^2*m_2^2*cos(y(3))^2 - L_1^2*l_2^2*m_2^3*cos(y(2))^2 - L_1^2*l_2^2*m_2^3*cos(y(3))^2 + l_1^2*l_2^2*m_0*m_1*m_2 - l_1^2*l_2^2*m_1^2*m_2*cos(y(2))^2 - l_1^2*l_2^2*m_1*m_2^2*cos(y(3))^2 - L_1^2*l_2^2*m_0*m_2^2*cos(y(2) - y(3))^2 - L_1^2*l_2^2*m_1*m_2^2*cos(y(2) - y(3))^2 - 2*L_1*l_1*l_2^2*m_1*m_2^2*cos(y(2))^2 + 2*L_1^2*l_2^2*m_2^3*cos(y(2) - y(3))*cos(y(2))*cos(y(3)) - 2*I_2*L_1*l_1*m_1*m_2*cos(y(2))^2 + 2*L_1*l_1*l_2^2*m_1*m_2^2*cos(y(2) - y(3))*cos(y(2))*cos(y(3))) + (g*l_2*m_2*sin(y(3))*(I_1*m_0 + I_1*m_1 + I_1*m_2 + L_1^2*m_2^2 + l_1^2*m_1^2 + l_1^2*m_0*m_1 + l_1^2*m_1*m_2 - L_1^2*m_2^2*cos(y(2))^2 - l_1^2*m_1^2*cos(y(2))^2 + L_1^2*m_0*m_2 + L_1^2*m_1*m_2 - 2*L_1*l_1*m_1*m_2*cos(y(2))^2))/(I_2*L_1^2*m_2^2 + I_2*l_1^2*m_1^2 + I_1*l_2^2*m_2^2 + I_1*I_2*m_0 + I_1*I_2*m_1 + I_1*I_2*m_2 + L_1^2*l_2^2*m_2^3 + L_1^2*l_2^2*m_0*m_2^2 + L_1^2*l_2^2*m_1*m_2^2 - L_1^2*l_2^2*m_2^3*cos(y(2) - y(3))^2 + I_2*L_1^2*m_0*m_2 + I_2*L_1^2*m_1*m_2 + l_1^2*l_2^2*m_1*m_2^2 + l_1^2*l_2^2*m_1^2*m_2 + I_2*l_1^2*m_0*m_1 + I_1*l_2^2*m_0*m_2 + I_1*l_2^2*m_1*m_2 + I_2*l_1^2*m_1*m_2 - I_2*L_1^2*m_2^2*cos(y(2))^2 - I_2*l_1^2*m_1^2*cos(y(2))^2 - I_1*l_2^2*m_2^2*cos(y(3))^2 - L_1^2*l_2^2*m_2^3*cos(y(2))^2 - L_1^2*l_2^2*m_2^3*cos(y(3))^2 + l_1^2*l_2^2*m_0*m_1*m_2 - l_1^2*l_2^2*m_1^2*m_2*cos(y(2))^2 - l_1^2*l_2^2*m_1*m_2^2*cos(y(3))^2 - L_1^2*l_2^2*m_0*m_2^2*cos(y(2) - y(3))^2 - L_1^2*l_2^2*m_1*m_2^2*cos(y(2) - y(3))^2 - 2*L_1*l_1*l_2^2*m_1*m_2^2*cos(y(2))^2 + 2*L_1^2*l_2^2*m_2^3*cos(y(2) - y(3))*cos(y(2))*cos(y(3)) - 2*I_2*L_1*l_1*m_1*m_2*cos(y(2))^2 + 2*L_1*l_1*l_2^2*m_1*m_2^2*cos(y(2) - y(3))*cos(y(2))*cos(y(3)));

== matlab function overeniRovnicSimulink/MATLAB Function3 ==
function dx = PohybovaRceDIP_simplified(y, u, g, m_1, m_2, I_1, I_2, l_1, l_2, L_1, b_1, b_2)
%PohybovaRceDIP_simplified: Zjednodusena pohybova rovnice dvojiteho kyvadla

dx = zeros(6, 1); % definovani sloupcoveho vektoru derivaci stavu 

dx(1) = conj(y(4)); 
dx(2) = conj(y(5)); 
dx(3) = conj(y(6)); 
dx(4) = u; 
dx(5) = conj(y(6))*(((I_2 + l_2^2*m_2)*(b_2 - L_1*l_2*m_2*sin(y(2) - y(3))*y(6)))/(I_1*I_2 + L_1^2*l_2^2*m_2^2 + I_2*L_1^2*m_2 + I_2*l_1^2*m_1 + I_1*l_2^2*m_2 - L_1^2*l_2^2*m_2^2*cos(y(2) - y(3))^2 + l_1^2*l_2^2*m_1*m_2) + (L_1*b_2*l_2*m_2*cos(y(2) - y(3)))/(I_1*I_2 + L_1^2*l_2^2*m_2^2 + I_2*L_1^2*m_2 + I_2*l_1^2*m_1 + I_1*l_2^2*m_2 - L_1^2*l_2^2*m_2^2*cos(y(2) - y(3))^2 + l_1^2*l_2^2*m_1*m_2)) - conj(y(5))*(((b_1 + b_2)*(I_2 + l_2^2*m_2))/(I_1*I_2 + L_1^2*l_2^2*m_2^2 + I_2*L_1^2*m_2 + I_2*l_1^2*m_1 + I_1*l_2^2*m_2 - L_1^2*l_2^2*m_2^2*cos(y(2) - y(3))^2 + l_1^2*l_2^2*m_1*m_2) + (L_1*l_2*m_2*cos(y(2) - y(3))*(b_2 + L_1*l_2*m_2*sin(y(2) - y(3))*y(5)))/(I_1*I_2 + L_1^2*l_2^2*m_2^2 + I_2*L_1^2*m_2 + I_2*l_1^2*m_1 + I_1*l_2^2*m_2 - L_1^2*l_2^2*m_2^2*cos(y(2) - y(3))^2 + l_1^2*l_2^2*m_1*m_2)) - (u*(L_1*l_2^2*m_2^2*cos(y(2)) + I_2*L_1*m_2*cos(y(2)) + I_2*l_1*m_1*cos(y(2)) - L_1*l_2^2*m_2^2*cos(y(2) - y(3))*cos(y(3)) + l_1*l_2^2*m_1*m_2*cos(y(2))))/(I_1*I_2 + L_1^2*l_2^2*m_2^2 + I_2*L_1^2*m_2 + I_2*l_1^2*m_1 + I_1*l_2^2*m_2 - L_1^2*l_2^2*m_2^2*cos(y(2) - y(3))^2 + l_1^2*l_2^2*m_1*m_2) + (g*sin(y(2))*(I_2 + l_2^2*m_2)*(L_1*m_2 + l_1*m_1))/(I_1*I_2 + L_1^2*l_2^2*m_2^2 + I_2*L_1^2*m_2 + I_2*l_1^2*m_1 + I_1*l_2^2*m_2 - L_1^2*l_2^2*m_2^2*cos(y(2) - y(3))^2 + l_1^2*l_2^2*m_1*m_2) - (L_1*g*l_2^2*m_2^2*cos(y(2) - y(3))*sin(y(3)))/(I_1*I_2 + L_1^2*l_2^2*m_2^2 + I_2*L_1^2*m_2 + I_2*l_1^2*m_1 + I_1*l_2^2*m_2 - L_1^2*l_2^2*m_2^2*cos(y(2) - y(3))^2 + l_1^2*l_2^2*m_1*m_2); 
dx(6) = conj(y(5))*(((b_2 + L_1*l_2*m_2*sin(y(2) - y(3))*y(5))*(I_1 + L_1^2*m_2 + l_1^2*m_1))/(I_1*I_2 + L_1^2*l_2^2*m_2^2 + I_2*L_1^2*m_2 + I_2*l_1^2*m_1 + I_1*l_2^2*m_2 - L_1^2*l_2^2*m_2^2*cos(y(2) - y(3))^2 + l_1^2*l_2^2*m_1*m_2) + (L_1*l_2*m_2*cos(y(2) - y(3))*(b_1 + b_2))/(I_1*I_2 + L_1^2*l_2^2*m_2^2 + I_2*L_1^2*m_2 + I_2*l_1^2*m_1 + I_1*l_2^2*m_2 - L_1^2*l_2^2*m_2^2*cos(y(2) - y(3))^2 + l_1^2*l_2^2*m_1*m_2)) - conj(y(6))*((b_2*(I_1 + L_1^2*m_2 + l_1^2*m_1))/(I_1*I_2 + L_1^2*l_2^2*m_2^2 + I_2*L_1^2*m_2 + I_2*l_1^2*m_1 + I_1*l_2^2*m_2 - L_1^2*l_2^2*m_2^2*cos(y(2) - y(3))^2 + l_1^2*l_2^2*m_1*m_2) + (L_1*l_2*m_2*cos(y(2) - y(3))*(b_2 - L_1*l_2*m_2*sin(y(2) - y(3))*y(6)))/(I_1*I_2 + L_1^2*l_2^2*m_2^2 + I_2*L_1^2*m_2 + I_2*l_1^2*m_1 + I_1*l_2^2*m_2 - L_1^2*l_2^2*m_2^2*cos(y(2) - y(3))^2 + l_1^2*l_2^2*m_1*m_2)) - (u*(L_1^2*l_2*m_2^2*cos(y(3)) + I_1*l_2*m_2*cos(y(3)) - L_1^2*l_2*m_2^2*cos(y(2) - y(3))*cos(y(2)) + l_1^2*l_2*m_1*m_2*cos(y(3)) - L_1*l_1*l_2*m_1*m_2*cos(y(2) - y(3))*cos(y(2))))/(I_1*I_2 + L_1^2*l_2^2*m_2^2 + I_2*L_1^2*m_2 + I_2*l_1^2*m_1 + I_1*l_2^2*m_2 - L_1^2*l_2^2*m_2^2*cos(y(2) - y(3))^2 + l_1^2*l_2^2*m_1*m_2) + (g*l_2*m_2*sin(y(3))*(I_1 + L_1^2*m_2 + l_1^2*m_1))/(I_1*I_2 + L_1^2*l_2^2*m_2^2 + I_2*L_1^2*m_2 + I_2*l_1^2*m_1 + I_1*l_2^2*m_2 - L_1^2*l_2^2*m_2^2*cos(y(2) - y(3))^2 + l_1^2*l_2^2*m_1*m_2) - (L_1*g*l_2*m_2*cos(y(2) - y(3))*sin(y(2))*(L_1*m_2 + l_1*m_1))/(I_1*I_2 + L_1^2*l_2^2*m_2^2 + I_2*L_1^2*m_2 + I_2*l_1^2*m_1 + I_1*l_2^2*m_2 - L_1^2*l_2^2*m_2^2*cos(y(2) - y(3))^2 + l_1^2*l_2^2*m_1*m_2);

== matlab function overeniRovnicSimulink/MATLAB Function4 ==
function y = fcn(u)
%#codegen

y = mod(u+pi,2*pi)-pi;

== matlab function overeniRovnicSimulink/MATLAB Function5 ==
function y = fcn(u)
%#codegen

y = mod(u+pi,2*pi)-pi;
